[IBIS Ver]  4.0
[File Name]  lpc32x0_tfbga296.ibs
[File Rev]  1.0
[Date]  Fri Aug 18 10:34:29 2006
[Source]  Package model from Ansoft Q3D Extractor 7.1.1
[Notes]   IO models Rev 0.20 IBIS Model Design Automation Generation
[Copyright]  NXP Semiconductors 2006,2007. All rights reserved.
|   LPC32x0_TFBGA296 (296 TFBGA package) IBIS Model
[Disclaimer]
| NXP Semiconductors warrants and represents that the IBIS models
| identified herein are owned by NXP Semiconductors (NXP).  The
| models provided are not warranted as fully representing all of the
| operating characteristics and specifications of the semiconductor
| products to which the models relate.  Moreover, unless there is a
| signed, written agreement to the contrary, these models are furnished
| on an "as is" basis without support or warranty of any kind, either
| expressed or implied, regarding the use thereof, and NXP
| specifically disclaims all implied warranties of merchantability and
| fitness of the models for any purpose.
| NXP does not assume any liability arising out of the application
| or use of these IBIS models including infringement of patents and
| copyrights, nor does NXP convey any license under its patents and
| copyrights or the rights of others.
| NXP provides IBIS models as a service to our customers.  You and
| your company shall not distribute, convey, sell, or give these models
| to anyone else without receiving prior written permission from
| NXP.
[Define Package Model]  TFBGA296
[Manufacturer]  NXP Semiconductors
[OEM]  NXP Semiconductors
[Description] Full package IBIS model.
| Model includes all substrate
| features e.g. vias, bondwires, metal interconnect,
| dielectrics and mold compound.
| AC simulation frequency:  100 MHz
[Number Of Pins]  237
[Pin Numbers]
|Pin Num   Terminal Name
U15   | U1:ADIN0:181
T14   | U1:ADIN1:180
V16   | U1:ADIN2:182
G14   | U1:DBGEN:97
L3   | U1:EMC_A_00_P1_0:288
L4   | U1:EMC_A_01_P1_1:287
M1   | U1:EMC_A_02_P1_2:286
M2   | U1:EMC_A_03_P1_3:282
M3   | U1:EMC_A_04_P1_4:279
N1   | U1:EMC_A_05_P1_5:278
N2   | U1:EMC_A_06_P1_6:275
N3   | U1:EMC_A_07_P1_7:274
M4   | U1:EMC_A_08_P1_8:271
P1   | U1:EMC_A_09_P1_9:268
P2   | U1:EMC_A_10_P1_10:267
P3   | U1:EMC_A_11_P1_11:266
N4   | U1:EMC_A_12_P1_12:265
R1   | U1:EMC_A_13_P1_13:264
R2   | U1:EMC_A_14_P1_14:263
L1   | U1:EMC_A_15_P1_15:290
K3   | U1:EMC_A_16_P1_16:291
K4   | U1:EMC_A_17_P1_17:292
K2   | U1:EMC_A_18_P1_18:293
K1   | U1:EMC_A_19_P1_19:296
J1   | U1:EMC_A_20_P1_20:297
J2   | U1:EMC_A_21_P1_21:298
J3   | U1:EMC_A_22_P1_22:301
J4   | U1:EMC_A_23_P1_23:302
U14   | U1:EMC_BLS_0:187
T13   | U1:EMC_BLS_1:186
R12   | U1:EMC_BLS_2:185
P12   | U1:EMC_BLS_3:184
R5   | U1:EMC_CAS_N:255
U3   | U1:EMC_CKE0:248
L2   | U1:EMC_CKE1:289
T3   | U1:EMC_CLK:250
T4   | U1:EMC_CLKIN:249
U13   | U1:EMC_CS0_N:193
R11   | U1:EMC_CS1_N:192
T12   | U1:EMC_CS2_N:190
V15   | U1:EMC_CS3_N:189
R3   | U1:EMC_DQM_0:262
P4   | U1:EMC_DQM_1:259
T1   | U1:EMC_DQM_2:258
P5   | U1:EMC_DQM_3:257
R6   | U1:EMC_DYCS0_N:253
G1   | U1:EMC_DYCS1_N:304
U4   | U1:EMC_D_00:246
R7   | U1:EMC_D_01:245
T5   | U1:EMC_D_02:244
U5   | U1:EMC_D_03:243
V3   | U1:EMC_D_04:242
V4   | U1:EMC_D_05:241
T6   | U1:EMC_D_06:238
R8   | U1:EMC_D_07:237
V5   | U1:EMC_D_08:236
U6   | U1:EMC_D_09:233
V6   | U1:EMC_D_10:232
T7   | U1:EMC_D_11:231
U7   | U1:EMC_D_12:229
V7   | U1:EMC_D_13:228
T8   | U1:EMC_D_14:227
U8   | U1:EMC_D_15:226
V8   | U1:EMC_D_16_DDR_DQS0:223
R9   | U1:EMC_D_17_DDR_DQS1:222
V9   | U1:EMC_D_18_DDR_NCLK:221
U9   | U1:EMC_D_19:220
T9   | U1:EMC_D_20:219
V10   | U1:EMC_D_21:214
U10   | U1:EMC_D_22:213
T10   | U1:EMC_D_23:209
R10   | U1:EMC_D_24:208
V11   | U1:EMC_D_25:207
U11   | U1:EMC_D_26:206
T11   | U1:EMC_D_27:203
V12   | U1:EMC_D_28:200
V13   | U1:EMC_D_29:199
U12   | U1:EMC_D_30:198
V14   | U1:EMC_D_31:196
H1   | U1:EMC_OE_N:303
T2   | U1:EMC_RAS_N:254
R4   | U1:EMC_WR_N:256
D2   | U1:FLASH_ALE:320
E3   | U1:FLASH_CE_N:325
F3   | U1:FLASH_CLE:328
H2   | U1:FLASH_IO_00:306
H3   | U1:FLASH_IO_01:307
F1   | U1:FLASH_IO_02:308
E1   | U1:FLASH_IO_03:309
H4   | U1:FLASH_IO_04:311
G2   | U1:FLASH_IO_05:312
G3   | U1:FLASH_IO_06:313
E2   | U1:FLASH_IO_07:314
D1   | U1:FLASH_RDY:319
C1   | U1:FLASH_RD_N:327
F2   | U1:FLASH_WR_N:326
A12   | U1:GPIO_00:48
A11   | U1:GPIO_01:47
D9   | U1:GPIO_02_KEY_ROW6_ENET_MDC:46
C11   | U1:GPIO_03_KEY_ROW7_ENET_MDIO:45
B11   | U1:GPIO_04_SSEL1_LCD_22:42
E9   | U1:GPIO_05_SSEL0:41
C16   | U1:GPI_00_ENET_RXD2:76
C15   | U1:GPI_01_SERVICE_N:75
C14   | U1:GPI_02_CAP2_0_ENET_RXD3:74
F4   | U1:GPI_03:330
E13   | U1:GPI_04_SPI1_BUSY:73
N16   | U1:GPI_05_U3_DCD:142
C7   | U1:GPI_06_HSTIM_CAP_I2SRX_SDA1:24
D13   | U1:GPI_07_PCAP3_0:72
B16   | U1:GPI_08_KEY_COL6_SPI2_BUSY_ENET_RX_DV:69
E12   | U1:GPI_09_KEY_COL7_ENET_COL:68
B15   | U1:GPI_10_U4_RX:67
N17   | U1:GPI_11_U3_RI:141
C3   | U1:GPO_00_TST_CLK1:337
D4   | U1:GPO_01:336
B14   | U1:GPO_02_MAT1_0_LCD_0:66
D12   | U1:GPO_03_LCD_1:65
D8   | U1:GPO_04:26
B3   | U1:GPO_05:335
A16   | U1:GPO_06_PWM4_3_LCD_18:64
A15   | U1:GPO_07_LCD_2:63
C13   | U1:GPO_08_PWM4_2_LCD_8:60
C12   | U1:GPO_09_PWM4_1_LCD_9:59
E11   | U1:GPO_10_PWM3_6_LCDPWR:58
E8   | U1:GPO_11:25
B12   | U1:GPO_12_PWM3_5_LCDLE:57
B13   | U1:GPO_13_PWM3_4_LCDCP:56
D3   | U1:GPO_14:334
A14   | U1:GPO_15_PWM3_3_LCDFP:55
D10   | U1:GPO_16_PWM3_2_LCDAC:54
N18   | U1:GPO_17:140
D11   | U1:GPO_18_PWM3_1_LCDLP:51
C2   | U1:GPO_19:333
B2   | U1:GPO_20:331
A13   | U1:GPO_21_U4_TX_LCD_3:50
E10   | U1:GPO_22_U7_HRTS_LCD_14:49
M16   | U1:GPO_23_U2_HRTS_U3_RTS:135
H16   | U1:HIGHCORE_LCD_17:107
A5   | U1:I2C1_SCL:20
B6   | U1:I2C1_SDA:21
A3   | U1:I2C2_SCL:338
E4   | U1:I2C2_SDA:339
A4   | U1:I2STX_CLK1_MAT3_0:11
E7   | U1:I2STX_SDA1_MAT3_1:12
B4   | U1:I2STX_WS1_CAP3_0:10
H17   | U1:JTAG_NTRST:113
H18   | U1:JTAG_RTCK:114
H14   | U1:JTAG_TCK:112
J16   | U1:JTAG_TDI:111
J15   | U1:JTAG_TDO:109
G18   | U1:JTAG_TMS:110
F15   | U1:KEY_COL0_ENET_TX_CLK:90
E16   | U1:KEY_COL1_ENET_RX_CLK_ENET_REF_CLK:91
D17   | U1:KEY_COL2_ENET_RX_ER:92
D18   | U1:KEY_COL3_ENET_CRS:94
G15   | U1:KEY_COL4_ENET_RXD0:95
F16   | U1:KEY_COL5_ENET_RXD1:96
E15   | U1:KEY_ROW0_ENET_TX_ER:82
E14   | U1:KEY_ROW1_ENET_TXD2:83
F14   | U1:KEY_ROW2_ENET_RXD3:86
D16   | U1:KEY_ROW3_ENET_TX_EN:87
C17   | U1:KEY_ROW4_ENET_TXD0:88
C18   | U1:KEY_ROW5_ENET_TXD1:89
A6   | U1:MS_BS_MAT2_1_PWM3_6:28
A8   | U1:MS_DIO0_MAT0_0_PWM3_1:32
A7   | U1:MS_DIO1_MAT0_1_PWM3_2:31
B8   | U1:MS_DIO2_MAT0_2_PWM3_3:30
C8   | U1:MS_DIO3_MAT0_3_PWM3_4:29
B7   | U1:MS_SCLK_MAT2_0_PWM3_5:27
M15   | U1:ONSW:146
B5   | U1:P0_0_I2SRX_CLK1:17
D7   | U1:P0_1_I2SRX_WS1:14
M17   | U1:P0_2_I2SRX_SDA0_LCD_4:134
M18   | U1:P0_3_I2SRX_CLK0_LCD_5:131
L15   | U1:P0_4_I2SRX_WS0_LCD_6:130
L16   | U1:P0_5_I2STX_SDA0_LCD_7:127
L17   | U1:P0_6_I2STX_CLK0_LCD_12:126
L18   | U1:P0_7_I2STX_WS0_LCD_13:123
R14   | U1:PLL397_LOOP:173
D14   | U1:PWM_OUT1_LCD_16:77
D15   | U1:PWM_OUT2_LCD_19:78
M14   | U1:RESET_N:147
G4   | U1:RESOUT_N:329
P16   | U1:RTCX_IN:152
P17   | U1:RTCX_OUT:151
C9   | U1:SPI1_CLK_SCK0:33
C10   | U1:SPI1_DATIN_MISO0:37
B9   | U1:SPI1_DATIO_MOSI0:34
B10   | U1:SPI2_CLK_SCK1_LCD_23:38
A10   | U1:SPI2_DATIN_MISO1_LCD_21:40
A9   | U1:SPI2_DATIO_MOSI1_LCD_20:39
G17   | U1:SYSCLKEN_LCD_15:108
T17   | U1:SYSX_IN:169
R15   | U1:SYSX_OUT:170
C6   | U1:TST_CLK2:13
R13   | U1:TS_XOUT:179
U16   | U1:TS_YOUT:177
K15   | U1:U1_RX_CAP1_0:121
K16   | U1:U1_TX:122
J18   | U1:U2_HCTS_U3_CTS:117
K18   | U1:U2_RX_U3_DSR:118
K17   | U1:U2_TX_U3_DTR:120
J14   | U1:U3_RX:115
J17   | U1:U3_TX:116
F18   | U1:U5_RX:105
H15   | U1:U5_TX:106
F17   | U1:U6_IRRX:103
G16   | U1:U6_IRTX:104
G13   | U1:U7_HCTS_CAP0_1_LCDCLKIN:98
E17   | U1:U7_RX_CAP0_0_LCD_10:99
E18   | U1:U7_TX_MAT1_1_LCD_11:100
C4   | U1:USB_ATX_INT_N:7
D5   | U1:USB_DAT_VP_U5_RX:3
E5   | U1:USB_I2C_SCL:340
E6   | U1:USB_I2C_SDA:2
D6   | U1:USB_OE_TP_N:6
C5   | U1:USB_SE0_VM_U5_TX:5
L12   | U1:VDD_COREFXD12:139
N14   | U1:VDD_FUSE:154
F8   | U1:VDD_IOB:15
T18   | U1:VDD_OSC12:168
T16   | U1:VDD_PLL397_12:172
R17   | U1:VDD_PLLHCLK_12:162
P15   | U1:VDD_PLLUSB_12:164
K14   | U1:VDD_RTC12:149
L13   | U1:VDD_RTCCORE12:143
N15   | U1:VDD_RTCOSC12:153
P13   | U1:VSS_AD:175
K13   | U1:VSS_IOA:129
F6   | U1:VSS_IOB:8
P14   | U1:VSS_OSC:171
T15   | U1:VSS_PLL397:174
R18   | U1:VSS_PLLHCLK:161
R16   | U1:VSS_PLLUSB:163
L14   | U1:VSS_RTCCORE:144
P18   | U1:VSS_RTCOSC:150
[Model Data]
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[End Model Data]
[End Package Model]
[Component]   LPC32x0_TFBGA296
[Manufacturer]  NXP
[Package]
|   typ   min   max
R_pkg   0   0   0  |Values included in package model
L_pkg   0   0   0  |Values included in package model
C_pkg   0   0   0  |Values included in package model
[Package Model]  TFBGA296
| (Pin and IO model definitions)
| IMPORTANT NOTES:
| This model is valid for the following part types:
| LPC3250
| LPC3240
| LPC3230
| LPC3220
[Pin]   signal_name   model_name   | comments
U15   ADIN0   NC   |apio3v3 not modeled
T14   ADIN1   NC   |apio3v3 not modeled
V16   ADIN2   NC   |apio3v3 not modeled
G14   DBGEN   bspts3chp
L3   EMC_A[00]/P1.0   mem1bsptz40pch
L4   EMC_A[01]/P1.1   mem1bsptz40pch
M1   EMC_A[02]/P1.2   mem1bsptz40pch
M2   EMC_A[03]/P1.3   mem1bsptz40pch
M3   EMC_A[04]/P1.4   mem1bsptz40pch
N1   EMC_A[05]/P1.5   mem1bsptz40pch
N2   EMC_A[06]/P1.6   mem1bsptz40pch
N3   EMC_A[07]/P1.7   mem1bsptz40pch
M4   EMC_A[08]/P1.8   mem1bsptz40pch
P1   EMC_A[09]/P1.9   mem1bsptz40pch
P2   EMC_A[10]/P1.10   mem1bsptz40pch
P3   EMC_A[11]/P1.11   mem1bsptz40pch
N4   EMC_A[12]/P1.12   mem1bsptz40pch
R1   EMC_A[13]/P1.13   mem1bsptz40pch
R2   EMC_A[14]/P1.14   mem1bsptz40pch
L1   EMC_A[15]/P1.15   mem1bsptz40pch
K3   EMC_A[16]/P1.16   mem1bsptz40pch
K4   EMC_A[17]/P1.17   mem1bsptz40pch
K2   EMC_A[18]/P1.18   mem1bsptz40pch
K1   EMC_A[19]/P1.19   mem1bsptz40pch
J1   EMC_A[20]/P1.20   mem1bsptz40pch
J2   EMC_A[21]/P1.21   mem1bsptz40pch
J3   EMC_A[22]/P1.22   mem1bsptz40pch
J4   EMC_A[23]/P1.23   mem1bsptz40pch
U14   EMC_BLS[0]   mem1bsptz40pch
T13   EMC_BLS[1]   mem1bsptz40pch
R12   EMC_BLS[2]   mem1bsptz40pch
P12   EMC_BLS[3]   mem1bsptz40pch
R5   EMC_CAS_N   mem1bsptz40pch
U3   EMC_CKE0   mem1bsptz40pch
L2   EMC_CKE1   mem1bsptz40pch
T3   EMC_CLK   mem1bsptz40pch
T4   EMC_CLKIN   mem1bsptz40pch
U13   EMC_CS0_N   mem1bsptz40pch
R11   EMC_CS1_N   mem1bsptz40pch
T12   EMC_CS2_N   mem1bsptz40pch
V15   EMC_CS3_N   mem1bsptz40pch
U4   EMC_D[00]   mem1bsptz40pch
R7   EMC_D[01]   mem1bsptz40pch
T5   EMC_D[02]   mem1bsptz40pch
U5   EMC_D[03]   mem1bsptz40pch
V3   EMC_D[04]   mem1bsptz40pch
V4   EMC_D[05]   mem1bsptz40pch
T6   EMC_D[06]   mem1bsptz40pch
R8   EMC_D[07]   mem1bsptz40pch
V5   EMC_D[08]   mem1bsptz40pch
U6   EMC_D[09]   mem1bsptz40pch
V6   EMC_D[10]   mem1bsptz40pch
T7   EMC_D[11]   mem1bsptz40pch
U7   EMC_D[12]   mem1bsptz40pch
V7   EMC_D[13]   mem1bsptz40pch
T8   EMC_D[14]   mem1bsptz40pch
U8   EMC_D[15]   mem1bsptz40pch
V8   EMC_D[16]/DDR_DQS0   mem1bsptz40pch
R9   EMC_D[17]/DDR_DQS1   mem1bsptz40pch
V9   EMC_D[18]/DDR_NCLK   mem1bsptz40pch
U9   EMC_D[19]   mem1bsptz40pch
T9   EMC_D[20]   mem1bsptz40pch
V10   EMC_D[21]   mem1bsptz40pch
U10   EMC_D[22]   mem1bsptz40pch
T10   EMC_D[23]   mem1bsptz40pch
R10   EMC_D[24]   mem1bsptz40pch
V11   EMC_D[25]   mem1bsptz40pch
U11   EMC_D[26]   mem1bsptz40pch
T11   EMC_D[27]   mem1bsptz40pch
V12   EMC_D[28]   mem1bsptz40pch
V13   EMC_D[29]   mem1bsptz40pch
U12   EMC_D[30]   mem1bsptz40pch
V14   EMC_D[31]   mem1bsptz40pch
R3   EMC_DQM[0]   mem1bsptz40pch
P4   EMC_DQM[1]   mem1bsptz40pch
T1   EMC_DQM[2]   mem1bsptz40pch
P5   EMC_DQM[3]   mem1bsptz40pch
R6   EMC_DYCS0_N   mem1bsptz40pch
G1   EMC_DYCS1_N   mem1bsptz40pch
H1   EMC_OE_N   mem1bsptz40pch
T2   EMC_RAS_N   mem1bsptz40pch
R4   EMC_WR_N   mem1bsptz40pch
D2   FLASH_ALE   mem1bsptz40pch
E3   FLASH_CE_N   mem1bsptz40pch
F3   FLASH_CLE   mem1bsptz40pch
H2   FLASH_IO[00]   mem1bsptz40pch
H3   FLASH_IO[01]   mem1bsptz40pch
F1   FLASH_IO[02]   mem1bsptz40pch
E1   FLASH_IO[03]   mem1bsptz40pch
H4   FLASH_IO[04]   mem1bsptz40pch
G2   FLASH_IO[05]   mem1bsptz40pch
G3   FLASH_IO[06]   mem1bsptz40pch
E2   FLASH_IO[07]   mem1bsptz40pch
C1   FLASH_RD_N   mem1bsptz40pch
D1   FLASH_RDY   mem1bsptz40pch
F2   FLASH_WR_N   mem1bsptz40pch
C16   GPI00/I2SRX_SDA1   bspts3chp
C15   GPI01/SERVICE_N   bspts3chp
C14   GPI02/CAP2.0/E_RXD3   bspts3chp
F4   GPI03   bspts3chp
E13   GPI04/SPI1_BUSY   bspts3chp
N16   GPI05/U3_DCD   bspts3chp
C7   GPI06/HSTIM_CAP/RXD2  bspts3chp
D13   GPI07/PCAP3.0   bspts3chp
B16   GPI08/KEY_COL6/SPI2   bspts3chp
E12   GPI09/KEY_COL7/E_COL  bspts3chp
B15   GPI10/U4_RX   bspts3chp
N17   GPI11/U3_RI   bspts3chp
A12   GPIO00   bspts3chp
A11   GPIO01   bspts3chp
D9   GPIO02/KEY_ROW6/EDC   bspts3chp
C11   GPIO03/KEY_ROW7/EDIO  bspts3chp
B11   GPIO04/SSEL1/LCDVD22  bspts3chp
E9   GPIO05/SSEL0   bspts3chp
C3   GPO00/TST_CLK1   bspts3cp
D4   GPO01   bspts3chp
B14   GPO02/MAT1.0/LCDVD0   bspts3chp
D12   GPO03/LCDVD[1]   bspts3chp
D8   GPO04   bspts3chp
B3   GPO05   bspts3cp
A16   GPO06/PWM4.3/LCDVD18  bspts3chp
A15   GPO07/LCDVD[2]   bspts3chp
C13   GPO08/PWM4.2/LCDVD8   bspts3chp
C12   GPO09/PWM4.1/LCDVD9   bspts3chp
E11   GPO10/PWM3.6/LCDPWR   bspts3chp
E8   GPO11   bspts3chp
B12   GPO12/PWM3.5/LCDLE   bspts3chp
B13   GPO13/PWM3.4/LCDDCLK  bspts3chp
D3   GPO14   bspts3chp
A14   GPO15/PWM3.3/LCDFP   bspts3chp
D10   GPO16/PWM3.2/LENAB   bspts3chp
N18   GPO17   bspts3chp
D11   GPO18/PWM3.1/LCDLP   bspts3chp
C2   GPO19   bspts3chp
B2   GPO20   bspts3cp
A13   GPO21/U4_TX/L3   bspts3chp
E10   GPO22/U7_HRTS/L14   bspts3cp
M16   GPO23/U2_HRTS/U3_RTS  bspts3cp
H16   HIGHCORE/LCDVD17   bspts3cp
A5   I2C1_SCL   iic3m4sclt5v_400k
B6   I2C1_SDA   iic3m4sdat5v_400k
A3   I2C2_SCL   iic3m4sclt5v_400k
E4   I2C2_SDA   iic3m4sdat5v_400k
A4   I2STX_CLK1/MAT3.0   bspts3chp
E7   I2STX_SDA1/MAT3.1   bspts3chp
B4   I2STX_WS1/CAP3.0   bspts3chp
H17   JTAG_NTRST   bspts3chp
H18   JTAG_RTCK   bspts1cp
H14   JTAG_TCK   bspts3cp
J16   JTAG_TDI   bspts3cp
J15   JTAG_TDO   bspts1cp
G18   JTAG_TMS   bspts3cp
F15   KEY_COL0/ENET_TX_CK   bspts3chp
E16   KEY_COL1/ENET_RX_CK   bspts3chp
D17   KEY_COL2/ENET_RX_ER   bspts3chp
D18   KEY_COL3/ENET_CRS   bspts3chp
G15   KEY_COL4/ENET_RXD0   bspts3chp
F16   KEY_COL5/ENET_RXD1   bspts3chp
E15   KEY_ROW0/ENET_TX_ER   bspts3chp
E14   KEY_ROW1/ENET_TXD2   bspts3chp
F14   KEY_ROW2/ENET_TXD3   bspts3chp
D16   KEY_ROW3/ENET_TX_EN   bspts3chp
C17   KEY_ROW4/ENET_TXD0   bspts3chp
C18   KEY_ROW5/ENET_TXD1   bspts3chp
A6   MS_BS/MT2.1/PWM3.6   bspts3cp
A8   MS_DIO0/MT0.0/PM3.1   bspts3cp
A7   MS_DIO1/MT0.1/PM3.2   bspts3cp
B8   MS_DIO2/MT0.2/PM3.3   bspts3cp
C8   MS_DIO3/MT0.3/PM3.4   bspts3cp
B7   MS_SCLK/MT2.0/PM3.5   bspts3cp
B17   NC   NC
U2   NC   NC
V17   NC   NC
M15   ONSW   bspts3chp1v2v
B5   P0.0/I2SRX_CLK1   bspts3chp
D7   P0.1/I2SRX_WS1   bspts3chp
M17   P0.2/I2SRX_SDA0/L4   bspts3chp
M18   P0.3/I2SRX_CLK0/L5   bspts3chp
L15   P0.4/I2SRX_WS0/L6   bspts3chp
L16   P0.5/I2STX_SDA0/L7   bspts3chp
L17   P0.6/I2STX_CLK0/L12   bspts3chp
L18   P0.7/I2STX_WS0/L13   bspts3chp
R14   PLL397_LOOP   NC   |apio3v3 Not Modeled
D14   PWM_OUT1/LC16   bspts3cp
D15   PWM_OUT2/LC19   bspts3cp
M14   RESET_N   ipchp1v2t1v8v
G4   RESOUT_N   bspts3cp
P16   RTCX_IN   NC   |apio3v3 Not Modeled
P17   RTCX_OUT   NC   |apio3v3 Not Modeled
C9   SPI1_CLK/SCK0   bspts1cp
C10   SPI1_DATIN/MISO0   bspts3cp
B9   SPI1_DATIO/MOSI0   bspts1cp
B10   SPI2_CLK/SCK1/L23   bspts1cp
A10   SPI2_DTIN/MISO1/L21   bspts3cp
A9   SPI2_DTIO/MOSI1/L20   bspts1cp
G17   SYSCLKEN/L15   bspts3chp
T17   SYSX_IN   NC   |apio3v3 Not Modeled
R15   SYSX_OUT   NC   |apio3v3 Not Modeled
R13   TS_XOUT   NC   |apio3v3 Not Modeled
U16   TS_YOUT   NC   |apio3v3 Not Modeled
C6   TST_CLK2   bspts1cp
K15   U1_RX/CAP1.0   bspts3chp
K16   U1_TX   bspts3cp
J18   U2_HCTS/U3_CTS   bspts3cp
K18   U2_RX/U3_DSR   bspts3cp
K17   U2_TX/U3_DTR   bspts3cp
J14   U3_RX   bspts3cp
J17   U3_TX   bspts3cp
F18   U5_RX   bspts3cp
H15   U5_TX   bspts3cp
F17   U6_IRRX   bspts3cp
G16   U6_IRTX   bspts3cp
G13   U7_HCTS/CAP0.1/LLKIN   bspts3cp
E17   U7_RX/CAP0.0/L10   bspts3cp
E18   U7_TX/MAT1.1/L11   bspts3cp
C4   USB_ATX_INT_N   bspts3cp
D5   USB_DAT_VP/U5_RX   bspts3cp
E5   USB_I2C_SCL   iic3m4sclt5v_400k
E6   USB_I2C_SDA   iic3m4sdat5v_400k
D6   USB_OE_TP_N   bspts3chp
C5   USB_SE0_VM/U5_TX   bspts3cp
L12   VDD_COREFXD   power
N14   VDD_FUSE   power
F8   VDD_IOB   power
T18   VDD_OSC12   power
T16   VDD_PLL397_12   power
R17   VDD_PLLHCLK_12   power
P15   VDD_PLLUSB_12   power
K14   VDD_RTC12   power
L13   VDD_RTCCORE12   power
N15   VDD_RTCOSC12   power
P13   VSS_AD   gnd
K13   VSS_IOA   gnd
F6   VSS_IOB   gnd
P14   VSS_OSC   gnd
T15   VSS_PLL397   gnd
R18   VSS_RTCOSC   gnd
R16   VSS_PLLUSB   gnd
L14   VSS_RTCCORE   gnd
P18   VSS_RTCOSC   gnd
[Model Selector] ipchp1v2t1v8v
ipchp1v2t1v8v_p   Plain input Mode (p1=0, p2=1)
ipchp1v2t1v8v_pd   Pull Down Mode (p1=1, p2=1)
ipchp1v2t1v8v_pu   Pull Up Mode (p1=0, p2=0)
ipchp1v2t1v8v_r   Repeater Mode (p1=1, p2=0)
[Model Selector] mem1bsptz40pch
m1bsptz40pchp_p_sh   Plain input Mode (p1=0, p2=1)
m1bsptz40pchp_p_sl   Plain input Mode (p1=0, p2=1)
m1bsptz40pchp_pd_sh   Pull Down Mode (p1=1, p2=1)
m1bsptz40pchp_pd_sl   Pull Down Mode (p1=1, p2=1)
m1bsptz40pchp_pu_sh   Pull Up Mode (p1=0, p2=0)
m1bsptz40pchp_pu_sl   Pull Up Mode (p1=0, p2=0)
m1bsptz40pchp_r_sh   Repeater Mode (p1=1, p2=0)
m1bsptz40pchp_r_sl   Repeater Mode (p1=1, p2=0)
[Model Selector] bspts3chp1v2v
bspts3chp1v2v_p   Plain input Mode (p1=0, p2=1)
bspts3chp1v2v_pd   Pull Down Mode (p1=1, p2=1)
bspts3chp1v2v_pu   Pull Up Mode (p1=0, p2=0)
bspts3chp1v2v_r   Repeater Mode (p1=1, p2=0)
| |   Rev 0.20 IBIS Model Design Automation Generation   |
| |   N O N - S I L I C O N   C O R R E L A T E D   |
| |   This IBIS [Model] is pre-Beta tactical support   |
| |  Note: this IBIS [Model] contains clamp curves generated   |
| |   through simulation which should not be relied upon   |
| E-Mail Support : helpdesk.ltg@philips.com
| WWW Support   : http://pww.ltg.sc.philips.com/cio
| Generated at   : Philips Semiconductors LTG/CIO-Nijmegen
| Workstation   : nyhc02
| Date/Time   : 2004 Nov 4 (Thu) 11:48:34
| Pcc090lp jliolib_p50 3.1
|   0.90 um 3.3V pad library
|   five level metal
|   dual oxide
|   single threshold voltage
|   nominal line mixed supply
|   parasitic extracted netlists
| Process block b5
| bspt16mchp
|   Bidirectional Pad 3v3
|   3state Output
|   Plain Input
|   CMOS
|   Programmable between
|   - (p1=0, p2=1) plain input
|   - (p1=0, p2=0) with Pull Up
|   - (p1=1, p2=1) with Pull Down
|   - (p1=1, p2=0) with Repeater
|   Characterized at Core 1.2V and I/O 3.3V
| Plain input Mode (p1=0, p2=1)
[Model Selector] bspts1cp
bspts1cp_p   Plain input Mode (p1=0, p2=1)
bspts1cp_pd   Pull Down Mode (p1=1, p2=1)
bspts1cp_pu   Pull Up Mode (p1=0, p2=0)
bspts1cp_r   Repeater Mode (p1=1, p2=0)
[Model Selector] bspts3chp
bspts3chp_p   Plain input Mode (p1=0, p2=1)
bspts3chp_pd   Pull Down Mode (p1=1, p2=1)
bspts3chp_pu   Pull Up Mode (p1=0, p2=0)
bspts3chp_r   Repeater Mode (p1=1, p2=0)
[Model Selector] bspts3cp
bspts3cp_p   Plain input Mode (p1=0, p2=1)
bspts3cp_pd   Pull Down Mode (p1=1, p2=1)
bspts3cp_pu   Pull Up Mode (p1=0, p2=0)
bspts3cp_r   Repeater Mode (p1=1, p2=0)
| Models and submodels in the file (30): iic3m4sclt5v_400k (I/O_open_drain), iic3m4sdat5v_400k (I/O_open_drain), ipchp1v2t1v8v_p (Input), ipchp1v2t1v8v_pd (Input), ipchp1v2t1v8v_pu (Input), ipchp1v2t1v8v_r (Input), m1bsptz40pchp_p_sh (I/O), m1bsptz40pchp_p_sl (I/O), m1bsptz40pchp_pd_sh (I/O), m1bsptz40pchp_pd_sl (I/O), m1bsptz40pchp_pu_sh (I/O), m1bsptz40pchp_pu_sl (I/O), m1bsptz40pchp_r_sh (I/O), m1bsptz40pchp_r_sl (I/O), bspts3chp1v2v_p (I/O), bspts3chp1v2v_pd (I/O), bspts3chp1v2v_pu (I/O), bspts3chp1v2v_r (I/O), bspts1cp_p (I/O), bspts1cp_pd (I/O), bspts1cp_pu (I/O), bspts1cp_r (I/O), bspts3chp_p (I/O), bspts3chp_pd (I/O), bspts3chp_pu (I/O), bspts3chp_r (I/O), bspts3cp_p (I/O), bspts3cp_pd (I/O), bspts3cp_pu (I/O), bspts3cp_r (I/O)
